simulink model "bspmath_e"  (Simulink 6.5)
settings: Solver=ode45  StartTime=0.0  StopTime=400.0  RelTol=1e-3
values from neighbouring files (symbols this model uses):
  amp = 1    [bspmath_ini.m]
  gain = -1    [bspmath_ini.m]    (also in bspparameter_ini_e.m = 10)

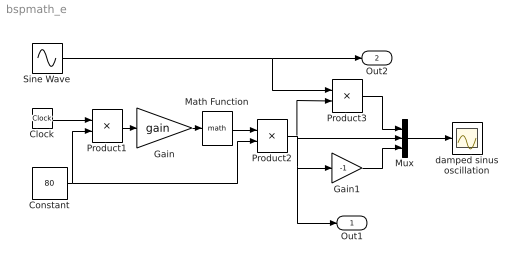
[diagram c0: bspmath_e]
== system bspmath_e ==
  Clock : Clock
  Constant : Constant  Value=80  OutDataType=sfix(16)  ConRadixGroup=Use specified scaling  OutScaling=2^0  SampleTime=inf  FramePeriod=inf
  Gain : Gain  Gain=gain
  Gain1 : Gain  Gain=-1
  Math Function : Math
  Mux : Mux  Inputs=3
  Product1 : Product  Inputs=*/
  Product2 : Product
  Product3 : Product
  Sine Wave : Sin  Amplitude=amp  Frequency=0.25  Phase=pi/3  SampleTime=0
  damped sinus oscillation : Scope
  Out1 : Outport
  Out2 : Outport  Port=2
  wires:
  Clock/1 -> Product1/1
  Product1/1 -> Gain/1
  Mux/1 -> damped sinus oscillation/1
  Constant/1 -> Product1/2, Product2/2
  Math Function/1 -> Product2/1
  Gain1/1 -> Mux/3
  Product2/1 -> Mux/2, Product3/2, Gain1/1, Out1/1
  Product3/1 -> Mux/1
  Gain/1 -> Math Function/1
  Sine Wave/1 -> Out2/1, Product3/1
